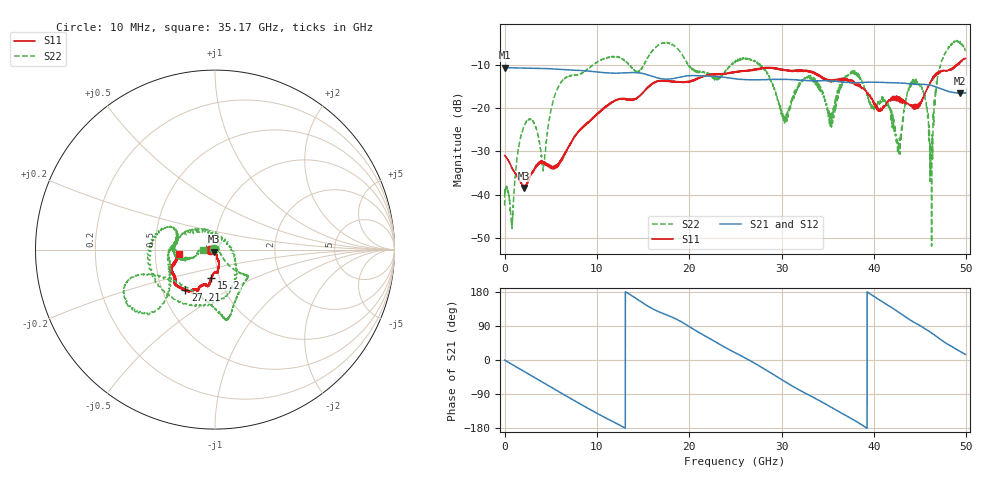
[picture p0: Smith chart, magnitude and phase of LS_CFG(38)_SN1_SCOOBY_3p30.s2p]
!Keysight Technologies,N5245B,MY58422026,A.13.80.08
!Date: Thursday, March 19, 2020 23:38:44
!Correction: S11(Full 2 Port(1,2))
!S21(Full 2 Port(1,2))
!S12(Full 2 Port(1,2))
!S22(Full 2 Port(1,2))
!S2P File: Measurements: S11, S21, S12, S22:
# Hz S DB R 50.0
!freq dBS11 angS11 dBS21 angS21 dBS12 angS12 dBS22 angS22
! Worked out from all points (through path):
!   4991 points, 10 MHz to 49.91 GHz, reference 50 ohm
!   highest |S21| = -10.61 dB at 10 MHz (marker M1); lowest = -16.5 dB at 49.34 GHz (marker M2)
!   group delay of S21, straight-line fit = 38.7 ps
!   lowest |S11| = -38.5 dB at 2.15 GHz (marker M3), VSWR 1.02, Z = 49.5 - j1.05 ohm
!   |S11| at or under -10 dB: start of sweep to 48.89 GHz; 48.93224 GHz to 48.99551 GHz (63.27 MHz wide, 0.129 % of centre); 49.07487 GHz to 49.08634 GHz (11.46 MHz wide, 0.0234 % of centre)
!   |S22| runs from -51.9 to -4.3 dB; largest |S21 - S12| = 0.0027
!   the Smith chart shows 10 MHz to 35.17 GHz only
!   S11 on the Smith chart (normalised r, x): 10 MHz: 0.95, -0.01; 15.2 GHz: 0.91, -0.29; 27.21 GHz: 0.65, -0.32; 35.17 GHz: 0.66, -0.03
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1e7  -30.94 -174.4  -10.61 -0.2  -10.60 -0.3  -42.56 171.6
8.2e8  -33.91 -172.7  -10.66 -11.8  -10.65 -11.8  -47.82 104.7
2.15e9  -38.48 -116.7  -10.73 -30.8  -10.72 -30.7  -24.04 54.0
4.19e9  -32.52 -86.4  -10.82 -59.6  -10.81 -59.6  -34.53 15.0
5.7e9  -33.38 -87.0  -10.99 -81.5  -10.98 -81.5  -15.63 -45.7
8.33e9  -24.88 -74.8  -11.30 -117.8  -11.29 -117.8  -11.94 -52.9
1.52e10  -16.06 -97.5  -12.11 147.0  -12.10 147.1  -9.60 -153.8
1.665e10  -13.79 -100.9  -13.04 127.9  -13.03 128.0  -5.42 -158.3
2.496e10  -11.71 -119.1  -13.18 19.3  -13.16 19.5  -9.40 168.3
2.721e10  -11.11 -126.6  -13.44 -10.3  -13.44 -10.1  -9.31 -117.8
3.036e10  -11.29 -143.9  -13.34 -56.8  -13.34 -56.6  -22.11 43.6
3.328e10  -11.61 -159.5  -13.63 -96.8  -13.63 -96.4  -12.89 -173.0
3.517e10  -13.84 -173.0  -13.65 -121.7  -13.59 -121.3  -23.17 -178.8
3.771e10  -14.19 168.3  -14.10 -156.8  -14.03 -157.0  -11.64 163.5
4.16e10  -18.13 103.5  -14.10 143.3  -14.12 143.2  -19.57 55.1
4.272e10  -18.40 98.4  -14.17 125.4  -14.20 125.3  -30.35 -2.4
4.378e10  -19.05 79.6  -14.32 107.9  -14.36 108.0  -15.55 -24.4
4.492e10  -18.96 34.1  -14.49 91.9  -14.51 91.9  -14.47 14.2
4.616e10  -13.77 9.4  -14.70 72.8  -14.72 72.9  -35.52 146.6
4.722e10  -11.44 8.4  -15.48 54.3  -15.49 54.3  -9.99 -88.9
4.934e10  -9.49 -17.5  -16.54 22.5  -16.56 22.7  -4.58 -32.4
4.991e10  -8.49 -15.4  -16.47 14.7  -16.50 14.7  -6.56 -20.2
